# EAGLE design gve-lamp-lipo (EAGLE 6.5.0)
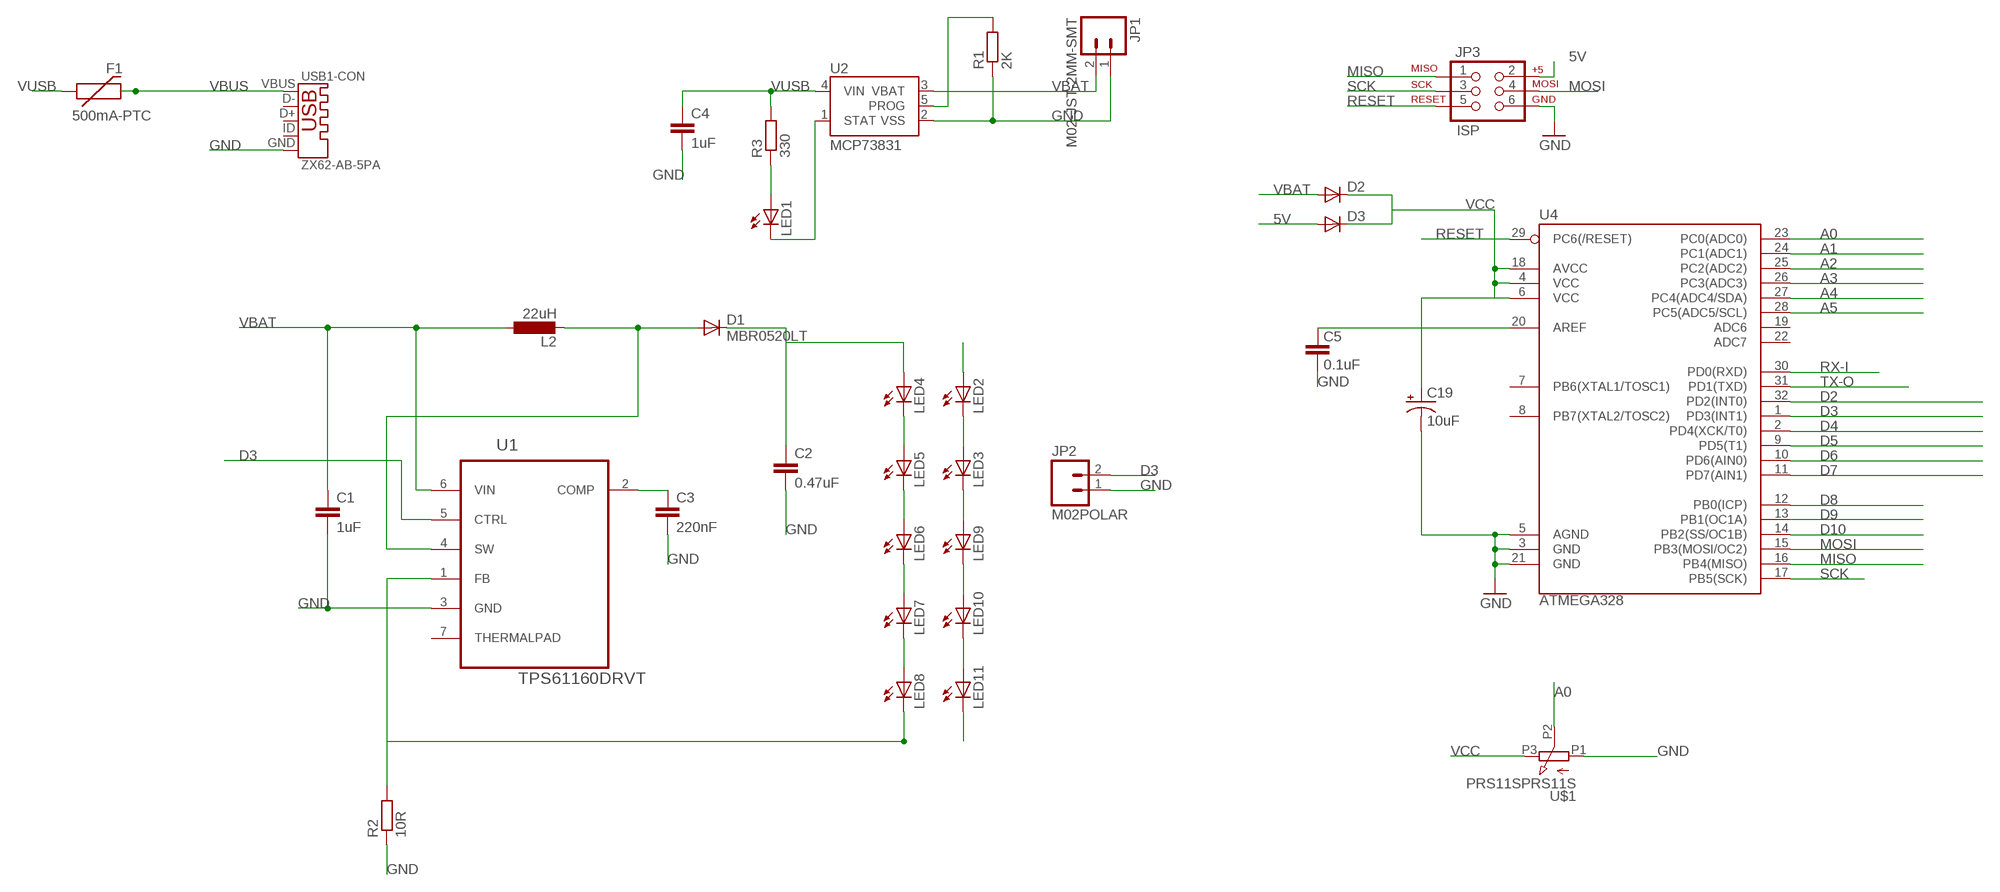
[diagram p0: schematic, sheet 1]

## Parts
C1  1uF  C-EUC0603K  [C0603K]
C2  0.47uF  C-EUC0603K  [C0603K]
C3  220nF  C-EUC0603K  [C0603K]
C4  1uF  C-EUC0603K  [C0603K]
C5  0.1uF  CAP0402-CAP  [0402-CAP]
C19  10uF  CAP_POL1206  [EIA3216]
D1  MBR0520LT  [SOD123]
D2  DIODESMA  [SMA-DIODE]
D3  DIODESMA  [SMA-DIODE]
F1  500mA-PTC  PTCSMD  [PTC-1206]
JP1  M02-JST-2MM-SMT  [JST-2-SMD]
JP2  M02POLAR  [MOLEX-1X2]
JP3  ISP  AVR_SPI_PRG_6PTH  [2X3]
L2  22uH  L-EUL5038P  [L5038P]
LED1  LED1206  [LED-1206]
LED2  LEDP-LCC-2  [P-LCC-2]
LED3  LEDP-LCC-2  [P-LCC-2]
LED4  LEDP-LCC-2  [P-LCC-2]
LED5  LEDP-LCC-2  [P-LCC-2]
LED6  LEDP-LCC-2  [P-LCC-2]
LED7  LEDP-LCC-2  [P-LCC-2]
LED8  LEDP-LCC-2  [P-LCC-2]
LED9  LEDP-LCC-2  [P-LCC-2]
LED10  LEDP-LCC-2  [P-LCC-2]
LED11  LEDP-LCC-2  [P-LCC-2]
R1  2K  R-EU_R1206  [R1206]
R2  10R  R-EU_R1206  [R1206]
R3  330  R-EU_R1206  [R1206]
U1  TPS61160DRVT  [SON65P210X210X80-7N]
U2  MCP73831  [SOT23-5]
U4  ATMEGA328  ATMEGA168  [TQFP32-08]
U$1  PRS11SPRS11S  [PRS11S]
USB1  ZX62-AB-5PA  [BOTTOM-MOUNT-SMT]

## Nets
5V: D3.A JP3.2
A0: U4.23(PC0(ADC0)) U$1.P2(S)
A1: U4.24(PC1(ADC1))
A2: U4.25(PC2(ADC2))
A3: U4.26(PC3(ADC3))
A4: U4.27(PC4(ADC4/SDA))
A5: U4.28(PC5(ADC5/SCL))
AREF: C5.2 U4.20(AREF)
D2: U4.32(PD2(INT0))
D3: JP2.2 U1.5(CTRL) U4.1(PD3(INT1))
D4: U4.2(PD4(XCK/T0))
D5: U4.9(PD5(T1))
D6: U4.10(PD6(AIN0))
D7: U4.11(PD7(AIN1))
D8: U4.12(PB0(ICP))
D9: U4.13(PB1(OC1A))
D10: U4.14(PB2(SS/OC1B))
GND: C1.2 C2.2 C3.2 C4.2 C5.1 C19.C(-) JP1.1 JP2.1 JP3.6 R1.1 R2.1 U1.3(GND) U2.2(VSS) U4.3(GND) U4.5(AGND) U4.21(GND) U$1.P1(A) USB1.5(-CON:GND)
MISO: JP3.1 U4.16(PB4(MISO))
MOSI: JP3.4 U4.15(PB3(MOSI/OC2))
N$1: C3.1 U1.2(COMP)
N$2: LED4.C LED5.A
N$3: LED2.C LED3.A
N$4: D1.A L2.2 U1.4(SW)
N$5: R1.2 U2.5(PROG)
N$6: LED1.A R3.1
N$7: LED5.C LED6.A
N$8: LED6.C LED7.A
N$9: LED7.C LED8.A
N$10: LED1.C U2.1(STAT)
N$11: LED3.C LED9.A
N$12: LED9.C LED10.A
N$13: LED10.C LED11.A
O0: LED8.C R2.2 U1.1(FB)
O1: LED11.C
RESET: JP3.5 U4.29(PC6(/RESET))
RX-I: U4.30(PD0(RXD))
SCK: JP3.3 U4.17(PB5(SCK))
TX-O: U4.31(PD1(TXD))
VBAT: C1.1 D2.A JP1.2 L2.1 U1.6(VIN) U2.3(VBAT)
VBUS: F1.2 USB1.1(-CON:VBUS)
VCC: C19.A(+) D2.C D3.C U4.4(VCC) U4.6(VCC) U4.18(AVCC) U$1.P3(E)
VUSB: C4.1 F1.1 R3.2 U2.4(VIN)
W: C2.1 D1.C LED4.A
W1: LED2.A
Unconnected: U1.7(THERMALPAD) U4.7(PB6(XTAL1/TOSC1)) U4.8(PB7(XTAL2/TOSC2)) U4.19(ADC6) U4.22(ADC7) USB1.2(-CON:D-) USB1.3(-CON:D+) USB1.4(-CON:ID) USB1.SHIELD1(-SHIELD1:SHIELD) USB1.SHIELD2(-SHIELD2:SHIELD) USB1.SHIELD3(-SHIELD3:SHIELD) USB1.SHIELD4(-SHIELD4:SHIELD) USB1.SHIELD5(-SHIELD5:SHIELD) USB1.SHIELD6(-SHIELD6:SHIELD)

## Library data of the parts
C1-C4 = rcl:C-EU: CAPACITOR, European symbol
C5 = SparkFun:CAP: Capacitor
C19 = SparkFun:CAP_POL: Capacitor Polarized
D1 = diode:MBR0520LT: SCHOTTKY BARRIER RECTIFIER
D2 D3 = SparkFun:DIODE: Diode
F1 = SparkFun:PTC: Resettable Fuse PTC
JP1 = SparkFun-Connectors:M02: Standard 2-pin 0.1" header. Use with; PROD_ID: CONN-08352
JP2 = SparkFun-Connectors:M02: Standard 2-pin 0.1" header. Use with
JP3 = SparkFun:AVR_SPI_PRG_6: AVR ISP 6 Pin This is the reduced ISP connector for AVR programming. Common on Arduino. This footprint will take up less PCB space and can be used with a 10-pin to 6-pin adapter such as SKU: BOB-08508
L2 = rcl:L-EU: INDUCTOR, European symbol
LED1 = SparkFun:LED: LEDs
LED2-LED11 = led:LED: LED
R1-R3 = rcl:R-EU_: RESISTOR, European symbol
U1 = Texas Instruments_By_element14_Batch_1:TPS61160DRVT: White LED Driver With Digital and PWM Brightness Control in 2mm x 2mm QFN Package for up to 10 LEDs in Series; MPN: TPS61160DRVT; OC_FARNELL: 1603420; OC_NEWARK: 65M6336; PACKAGE: SON-6; SUPPLIER: Texas Instruments
U2 = SparkFun:MCP73831: Microchip's MCP73831 Miniature single cell, fully integrated Li-Ion, Li-polymer charge management controller http://ww1.microchip.com/downloads/en/DeviceDoc/21984a.pdf
U4 = SparkFun:ATMEGA168; VALUE: ATMEGA328P
U$1 = Bourns_PRS11S:PRS11S
USB1 = con-hirose-zx:ZX62: Micro-USB Receptacle Extremely small high reliability connectors complying with physical, electrical and environmental requirements of Micro-USB standard (USB 2.0). Receptacles and plugs are available in a wide variety of mounting and termination configurations, permitting their use in various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

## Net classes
1 vcc: width 0.254 mm

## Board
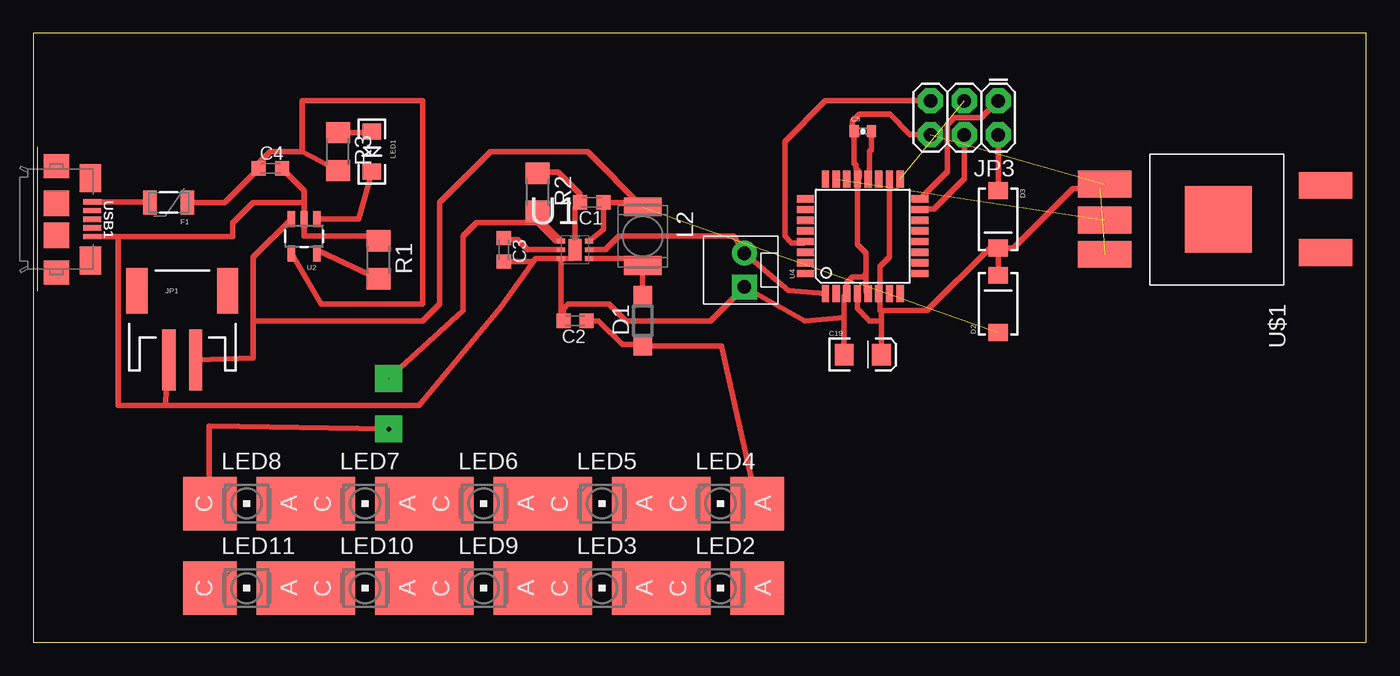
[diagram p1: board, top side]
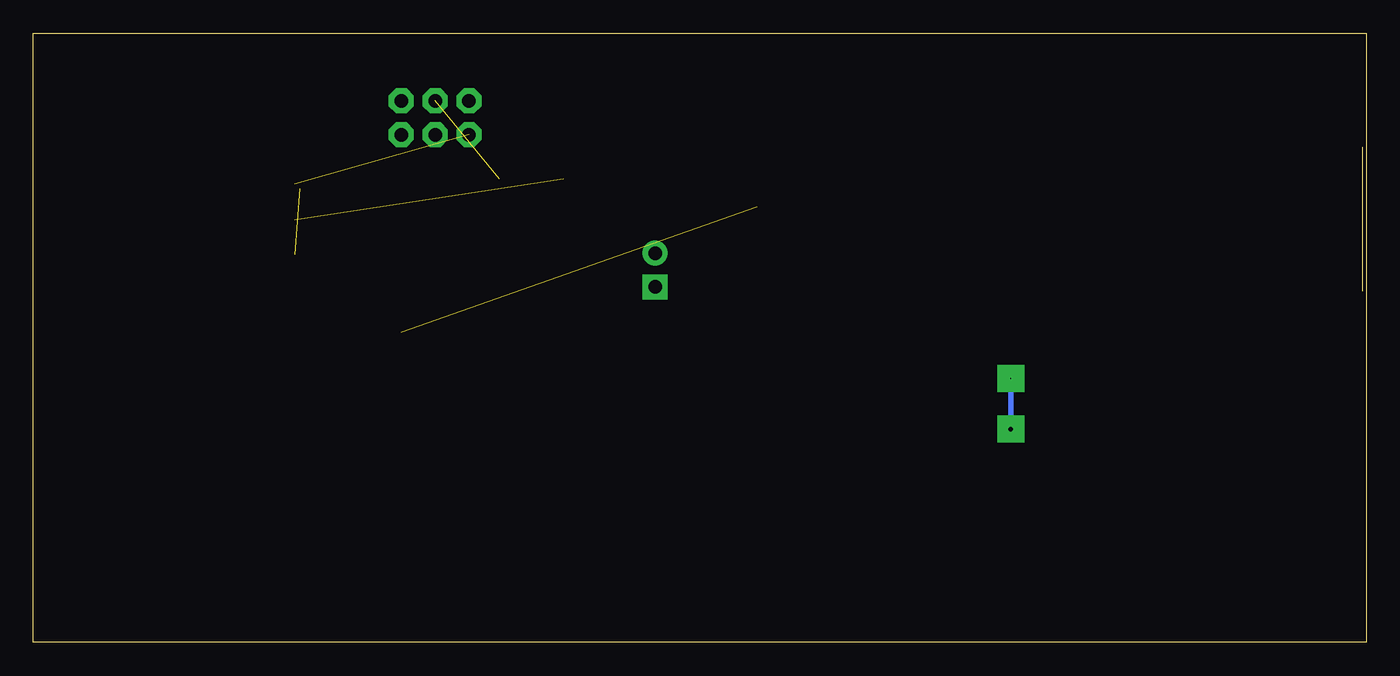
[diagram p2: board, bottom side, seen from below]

Size 100 x 45.71 mm. Coordinates in mm from the lower left corner, seen from the top.
Outline: 0,0 100,0 100,45.71 0,45.71 0,0
Copper layers (1*16): Top 0.035mm / dielectric 1.5mm / Bottom 0.035mm
Design rules "default": minimum track width 10mil, minimum drill 24mil, track to track 8mil, track to pad 8mil, pad to pad 8mil, via to via 8mil, smd to smd 8mil, copper to edge 40mil, drill to drill 8mil, minimum pad ring 10mil, minimum via ring 8mil, stop-mask expansion 4mil, vias tented up to drill 0mil, thermal gap 10mil

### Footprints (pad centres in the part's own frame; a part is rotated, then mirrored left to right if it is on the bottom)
C0603K = smd 1.05 x 1.08: 1 -0.875,0; 2 0.875,0
0402-CAP = smd 0.7 x 0.9: 1 -0.65,0; 2 0.65,0
EIA3216 = smd 1.4 x 1.6: A 1.4,0; C -1.4,0
SOD123 = smd 1.4 x 1.4: A 1.9,0; C -1.9,0
SMA-DIODE = smd 1.27 x 1.47: A -2.15,0; C 2.15,0
PTC-1206 = smd 1 x 1.8: 1 -1.4,0; 2 1.4,0
JST-2-SMD = smd 1 x 4.6: 1 -1,-3.7; 2 1,-3.7 | smd 1.6 x 3.4: NC1 -3.4,1.5; NC2 3.4,1.5
MOLEX-1X2 = drill 1.016 pad 1.88 square: 1 0,0 | drill 1.016 pad 1.88: 2 2.54,0
2X3 = drill 1.016 pad 1.88 octagon: 1 0,0; 2 0,2.54; 3 2.54,0; 4 2.54,2.54; 5 5.08,0; 6 5.08,2.54
L5038P = smd 1.4 x 2.8: 1 -2.2,0; 2 2.2,0
LED-1206 = smd 1.2 x 1.4: A -1.5,0; C 1.5,0
P-LCC-2 = smd 4 x 4: A 0,2.75; C 0,-2.75
R1206 = smd 1.6 x 1.803: 1 -1.422,0; 2 1.422,0
SON65P210X210X80-7N = smd 0.61 x 0.356: 1 -1.041,0.66; 2 -1.041,0; 3 -1.041,-0.66; 4 1.041,-0.66; 5 1.041,0; 6 1.041,0.66 | smd 0.991 x 1.6: 7 0,0
SOT23-5 = smd 0.55 x 1.2: 1 -0.95,-1.3; 2 0,-1.3; 3 0.95,-1.3; 4 0.95,1.3; 5 -0.95,1.3
TQFP32-08 = smd 1.27 x 0.559: 1 -4.293,2.8; 2 -4.293,2; 3 -4.293,1.2; 4 -4.293,0.4; 5 -4.293,-0.4; 6 -4.293,-1.2; 7 -4.293,-2; 8 -4.293,-2.8; 17 4.293,-2.8; 18 4.293,-2; 19 4.293,-1.2; 20 4.293,-0.4; 21 4.293,0.4; 22 4.293,1.2; 23 4.293,2; 24 4.293,2.8 | smd 0.559 x 1.27: 9 -2.8,-4.293; 10 -2,-4.293; 11 -1.2,-4.293; 12 -0.4,-4.293; 13 0.4,-4.293; 14 1.2,-4.293; 15 2,-4.293; 16 2.8,-4.293; 25 2.8,4.293; 26 2,4.293; 27 1.2,4.293; 28 0.4,4.293; 29 -0.4,4.293; 30 -1.2,4.293; 31 -2,4.293; 32 -2.8,4.293
PRS11S = smd 5 x 5: BOTTOM 0,0 | smd 2 x 4: P1 -2.64,-8.52; P2 0.06,-8.52; P3 2.63,-8.52; P4 -2.54,8.05; P5 2.5,8.05
BOTTOM-MOUNT-SMT = smd 0.4 x 1.35: 1 -1.3,-0.675; 2 -0.65,-0.675; 3 0,-0.675; 4 0.65,-0.675; 5 1.3,-0.675 | smd 2.1 x 1.6: SHIELD1 3.1,-0.8; SHIELD2 -3.1,-0.8 | smd 1.8 x 1.9: SHIELD3 4,-3.35; SHIELD6 -4,-3.35 | smd 1.9 x 1.9: SHIELD4 1.2,-3.35; SHIELD5 -1.2,-3.35

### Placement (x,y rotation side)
C1  41.91,33.02 180 top
C2  40.64,24.13 180 top
C3  35.31,29.46 270 top
C4  17.78,35.56 0 top
C5  62.23,38.35 0 top
C19  62.23,21.59 0 top
D1  45.72,24.13 90 top
D2  72.39,25.4 90 top
D3  72.39,31.75 270 top
F1  10.16,33.02 180 top
JP1  11.18,24.89 0 top
JP2  53.34,26.67 90 top
JP3  72.39,40.64 180 top
L2  45.72,30.48 270 top
LED1  25.4,36.83 270 top
LED2  51.56,4.06 270 top
LED3  42.67,4.06 270 top
LED4  51.56,10.41 270 top
LED5  42.67,10.41 270 top
LED6  33.78,10.41 270 top
LED7  24.89,10.41 270 top
LED8  16,10.41 270 top
LED9  33.78,4.06 270 top
LED10  24.89,4.06 270 top
LED11  16,4.06 270 top
R1  25.91,28.7 270 top
R2  37.85,33.78 270 top
R3  22.86,36.83 270 top
U1  40.64,29.46 0 top
U2  20.32,30.48 180 top
U4  62.23,30.48 90 top
U$1  88.9,31.75 270 top
USB1  5.08,31.75 270 top

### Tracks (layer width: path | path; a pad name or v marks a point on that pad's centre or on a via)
5V
  Top 0.406: JP3.2 D3.A
A0  (1 unrouted)
AREF
  Top 0.406: C5.2 62.88,36.97 62.74,36.83 62.74,34.88 U4.20
D3
  Top 0.406: U1.5 42.93,29.46 43.94,30.48 52.58,30.48 JP2.2 56.64,26.42 U4.1
GND  (1 unrouted)
  Top 0.406: USB1.5 6.35,30.45 | 6.35,30.45 14.97,30.45 14.97,31.48 16.51,33.02 20.32,33.02 | 20.32,33.02 U2.2 20.32,30.48 25.4,30.48 R1.1 | 20.32,33.02 20.32,33.9 C4.2 | U1.3 37.69,28.8 37.61,28.69 | 37.61,28.69 35.05,25.15 28.96,17.78 9.91,17.78 | 9.91,17.78 6.35,17.78 6.35,30.45 | C3.2 37.51,28.59 37.61,28.69 | R2.1 37.95,35.31 39.37,35.31 41.03,33.64 C1.2 40.64,32.62 40.64,29.46 40.49,28.8 U1.3 | U1.3 39.6,24.3 C2.2 39.77,25.03 40.13,25.4 43.18,25.4 44.45,24.13 50.8,24.13 JP2.1 57.91,24.13 60.83,24.38 | C19.C 60.83,24.38 | 60.83,24.38 60.83,25.99 U4.3 61.03,26.99 61.47,27.43 62.23,27.43 62.48,27.69 | 62.48,27.69 62.48,29.21 61.83,29.86 U4.21 61.98,34.92 61.98,35.31 61.72,35.56 61.72,35.81 61.58,35.96 C5.1 61.47,38.47 61.47,39.12 61.98,39.62 64.26,39.62 65.79,38.1 JP3.6 | 62.48,27.69 62.48,26.33 U4.5 | JP1.1 9.91,17.78
MISO
  Top 0.406: JP3.1 71.12,39.37 69.09,39.37 68.58,38.86 68.58,35.34 U4.16
MOSI
  Top 0.406: JP3.4 69.85,34.8 67.56,32.51 66.56,32.51 U4.15
N$1
  Top 0.406: U1.2 37.08,29.46 36.32,30.23 35.42,30.23 C3.1
N$2
  Top 0.406: LED5.A LED4.C
N$3
  Top 0.406: LED2.C LED3.A
N$4
  Top 0.406: U1.4 45.2,28.8 L2.2 D1.A
N$5
  Top 0.406: R1.2 21.45,29.36 U2.5
N$6
  Top 0.406: R3.1 25.32,38.25 LED1.A
N$7
  Top 0.406: LED6.A LED5.C 40.64,10.41
N$8
  Top 0.406: LED7.A 30.48,10.16 LED6.C
N$9
  Top 0.406: LED8.A LED7.C
N$10
  Top 0.406: U2.1 24.39,31.78 LED1.C
N$11
  Top 0.406: LED3.C LED9.A
N$12
  Top 0.406: LED9.C LED10.A
N$13
  Top 0.406: LED10.C 18.29,3.81 LED11.A
O0  (via drill 0.06 pad 2.03, 0.35 pad 2.03)
  Top 0.406: R2.2 37.85,31.88 U1.1 39.22,30.12 37.85,31.5 33.27,31.5 32.26,30.48 32.26,24.89 v26.67,19.81 | v26.67,16 13.21,16.26 13.21,12.45 LED8.C
  Bottom 0.406: v26.67,19.81 v26.67,16
RESET
  Top 0.406: JP3.5 59.44,40.64 56.39,37.59 56.39,30.48 56.9,29.97 57.83,29.97 U4.29
SCK  (1 unrouted)
VBAT  (1 unrouted)
  Top 0.406: 16.51,24.13 16.51,23.88 16.51,21.34 JP1.2 | 16.51,24.13 16.51,28.92 U2.3 | U1.6 42.78,30.97 C1.1 45.38,33.02 L2.1 41.57,36.83 34.29,36.83 30.48,33.02 30.48,25.4 29.21,24.13 16.51,24.13
VBUS
  Top 0.406: USB1.1 8.76,33.05 F1.2
VCC  (1 unrouted)
  Top 0.406: D3.C D2.C | C19.A 63.63,24.13 | 63.63,24.13 63.63,24.76 | 63.63,24.76 63.5,24.89 63.5,26.12 U4.6 63.5,26.26 63.5,28.19 64.23,28.92 U4.18 | U4.4 61.83,25.04 62.74,24.13 63.63,24.13 | D3.C 71.76,29.6 67.06,24.89 63.76,24.89 63.63,24.76 | D3.C 73.54,29.6 77.98,34.04 80.03,34.04
VUSB
  Top 0.406: F1.1 14.37,33.02 C4.1 16.91,35.95 17.78,36.83 20.17,36.83 | 20.17,36.83 R3.2 | U2.4 21.59,25.4 29.21,25.4 29.21,40.64 20.17,40.64 20.17,36.83
W
  Top 0.406: C2.1 42.42,24.13 44.2,22.35 45.6,22.35 D1.C 51.64,22.23 LED4.A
